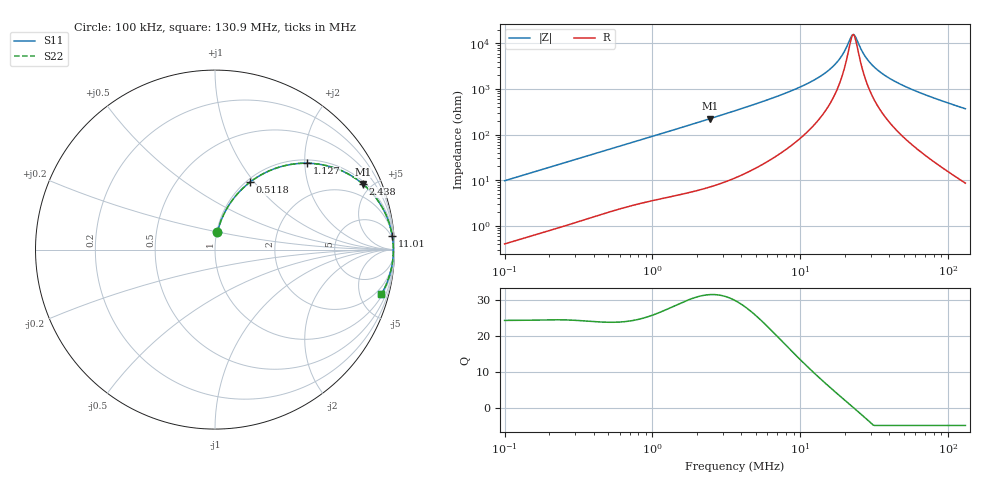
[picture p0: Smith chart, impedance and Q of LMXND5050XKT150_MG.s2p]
! LMXND5050XKT150_MG  S-PARAMETER MODEL  ( General Type )
! Model Generated by TAIYO YUDEN Corporation (http://www.ty-top.com)
! Version 1.0
! TAIYO YUDEN Control No. 191023NI43SB-FBB
! Copyright(c) 2019 TAIYO YUDEN CO.,LTD. All Rights Reserved.
! Product Description (link to TY-COMPAS)
! https://ds.yuden.co.jp/TYCOMPAS/or/detail?pn=LMXND5050XKT150MMG&u=M
! Products Name : Inductors
! Characteristics :
!  Inductance : 15 uH , SRF(min) : 14 MHz , DC Resistance(max) : 0.1625 Ohm
!  Rated Current : Saturation :1600 mA , Temp Rise : 1400 mA
!  Case Size : 4.9 x 4.9 / 0.193 x 0.193 [mm/inch] , Thickness : 3 / 0.118 [mm/inch]
!  (Conditions: Temperature = 25 degC , DC Bias Current/Voltage = 0A / 0V)
! External Node Assignments :
!  1  o---GGG---o  2
! GND o---------o GND
! Frequency Range : 0.1MHz  -  130.914307MHz  [ 402 STEP ]
# MHz S RI R 50
! Freq[MHz].  S11 Real  S11 Imag  S21 Real  S21 Imag  S12 Real  S12 Imag  S22 Real  S22 Imag
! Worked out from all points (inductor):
!   401 points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, 100 kHz to 130.9 MHz, reference 50 ohm
!   read as one part in series: L = 15.4 uH near 103.7 kHz
!   highest Q = 31.4 at 2.438 MHz (marker M1), where L = 14.5 uH
!   self-resonance near 22.56 MHz
!   S11 on the Smith chart (normalised r, x): 100 kHz: 1.01, +0.19; 511.8 kHz: 1.04, +0.96; 1.127 MHz: 1.08, +2.06; 2.438 MHz: 1.14, +4.44; 11.01 MHz: 3, +26; 130.9 MHz: 1.17, -7.37
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0.1  0.0132 0.0956  0.9868 -0.0956  0.9868 -0.0956  0.0132 0.0956
0.332733  0.0995 0.2794  0.9005 -0.2794  0.9005 -0.2794  0.0995 0.2794
0.511817  0.196 0.3765  0.804 -0.3765  0.804 -0.3765  0.196 0.3765
1.10711  0.5061 0.4814  0.4939 -0.4814  0.4939 -0.4814  0.5061 0.4814
1.127154  0.5146 0.4813  0.4854 -0.4813  0.4854 -0.4813  0.5146 0.4813
2.438144  0.824 0.3652  0.176 -0.3652  0.176 -0.3652  0.824 0.3652
3.683715  0.9129 0.2657  0.0871 -0.2657  0.0871 -0.2657  0.9129 0.2657
7.027727  0.9731 0.1385  0.0269 -0.1385  0.0269 -0.1385  0.9731 0.1385
11.00592  0.9875 0.0762  0.0125 -0.0762  0.0125 -0.0762  0.9875 0.0762
12.03896  0.9891 0.0656  0.0109 -0.0656  0.0109 -0.0656  0.9891 0.0656
14.66581  0.9916 0.044  0.00839 -0.044  0.00839 -0.044  0.9916 0.044
17.23607  0.9929 0.0274  0.00714 -0.0274  0.00714 -0.0274  0.9929 0.0274
19.54274  0.9934 0.0151  0.00657 -0.0151  0.00657 -0.0151  0.9934 0.0151
22.15811  0.9937 0.0029  0.00632 -0.0029  0.00632 -0.0029  0.9937 0.0029
22.96771  0.9937 -0.000559  0.0063 0.000559  0.0063 0.000559  0.9937 -0.000559
23.80689  0.9937 -0.00402  0.00631 0.00402  0.00631 0.00402  0.9937 -0.00402
26.99292  0.9935 -0.0162  0.00654 0.0162  0.00654 0.0162  0.9935 -0.0162
29.52652  0.9931 -0.025  0.0069 0.025  0.0069 0.025  0.9931 -0.025
33.478  0.9923 -0.0377  0.00769 0.0377  0.00769 0.0377  0.9923 -0.0377
40.05754  0.9905 -0.0569  0.00951 0.0569  0.00951 0.0569  0.9905 -0.0569
65.02508  0.9794 -0.1185  0.0206 0.1185  0.0206 0.1185  0.9794 -0.1185
130.9143  0.9264 -0.2496  0.0736 0.2496  0.0736 0.2496  0.9264 -0.2496
